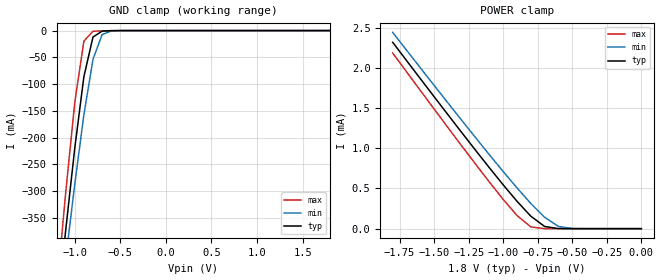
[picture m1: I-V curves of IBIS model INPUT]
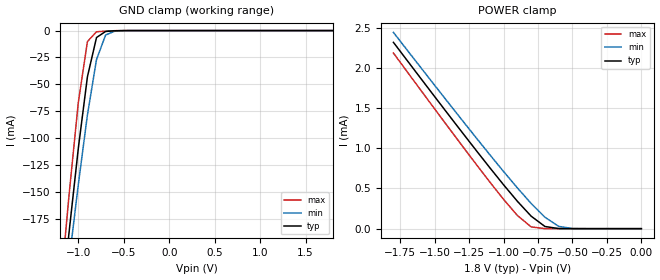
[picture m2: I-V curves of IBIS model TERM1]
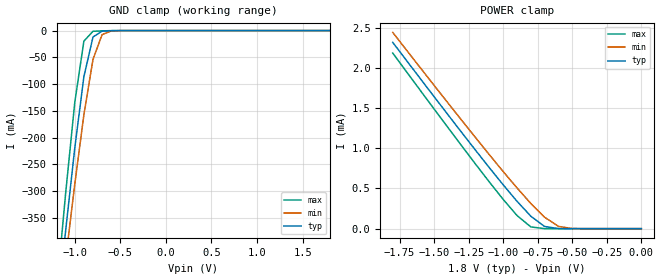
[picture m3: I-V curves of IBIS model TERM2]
|   PERICOM SEMICONDUCTOR CORP
|   IBIS Model of PI4MSD5V9545A
|   Product Family: 4MSD
|   TSSOP-20 (L) Package
[IBIS Ver] 3.2
[Comment char] |_char
[File Name] pi4msd5v9545a_l_18v.ibs
[File Rev] 1.0
[Source] File originated at Pericom Semiconductor Corp.
[Date] 09/07/17
[Disclaimer] (C) Copyright PERICOM Semiconductor Corporation
   All rights reserved
  Pericom Semiconductor Corporation hereby grants the user of
  this IBIS model a non-exclusive, nontransferable license to
  use this IBIS model under the following terms.
  This IBIS model is provided on an "AS IS" basis and Pericom
  makes absolutely no warranty with respect to the information
  contained herein. PERICOM DISCLAIMS AND CUSTOMER WAIVES ALL
  WARRANTIES, EXPRESSED OR IMPLIED, INCLUDING WARRANTIES OF
  MERCHANTABILITY OR FITNESS FOR A PARTICULAR PURPOSE. The
  entire risk as to quality and performance is with the customer.
  Accordingly, in no event shall the company be liable for any
  damages, whether in contract or tort, including any lost
  profits or other incidental, consequential, exemplary, or
  punitive damages arising out of the use or application of the
  IBIS model provided in this package. Further, Pericom reserves
  the right to make changes without notice to any product herein
  to improve reliability, function, or design. Pericom does not
  convey any license under patent rights or any other intellectual
  property rights, including those of third parties.
  The user is granted this license only to use the IBIS model
  and is not granted rights to sell, load, rent, lease or license
  the IBIS model in whole or in part, or in modified form to anyone
  other than user. User may modify the IBIS model to suit its specific
  application but rights to derivative works and such modifications
  shall belong to Pericom.
  Pericom is not obligated to provide maintenance or support
  for the licensed IBIS model.
  Contact Pericom at ATTN: APPLICATION ENGINEERING / IBIS MODELS
  2380 Bering Drive, San Jose, CA 95131
[Component] PI4MSD5V9545A
[Manufacturer] Pericom Semiconductor Corp.
[Package]
| variable   typ   min   max
R_pkg   0.03869ohm   0.03668ohm   0.04069ohm
L_pkg   2.64482nH   2.06962nH   3.22001nH
C_pkg   0.19279pF   0.15543pF   0.23014pF
[Pin] signal_name   model_name   R_pin   L_pin   C_pin
1   A0   INPUT   0.04069   3.22001nH   0.23014pF
2   A1   INPUT   0.03969   2.93241nH   0.21146pF
3   _RESET   INPUT   0.03869   2.64482nH   0.19279pF
4   _INT0   INPUT   0.03768   2.35722nH   0.17411pF
5   SD0   TERM1   0.03668   2.06962nH   0.15543pF
6   SC0   TERM1   0.03668   2.06962nH   0.15543pF
7   _INT1   INPUT   0.03768   2.35722nH   0.17411pF
8   SD1   TERM1   0.03869   2.64482nH   0.19279pF
9   SC1   TERM1   0.03969   2.93241nH   0.21146pF
10   GND   GND   0.04069   3.22001nH   0.23014pF
11   _INT2   INPUT   0.04069   3.22001nH   0.23014pF
12   SD2   TERM1   0.03969   2.93241nH   0.21146pF
13   SC2   TERM1   0.03869   2.64482nH   0.19279pF
14   _INT3   INPUT   0.03768   2.35722nH   0.17411pF
15   SD3   TERM1   0.03668   2.06962nH   0.15543pF
16   SC3   TERM1   0.03668   2.06962nH   0.15543pF
17   _INT   INPUT   0.03768   2.35722nH   0.17411pF
18   SCL   TERM2   0.03869   2.64482nH   0.19279pF
19   SDA   TERM2   0.03969   2.93241nH   0.21146pF
20   VCC   POWER   0.04069   3.22001nH   0.23014pF
[Series Switch Groups]
On 1 /
Off 2 3 4 /
[Series Pin Mapping]   pin_2   model_name  function_table_group
6   18   SWITCH1   1
5   19   SWITCH1   1
9   18   SWITCH1   2
8   19   SWITCH1   2
13   18   SWITCH1   3
12   19   SWITCH1   3
16   18   SWITCH1   4
15   19   SWITCH1   4
|   Model SWITCH1
[Model] SWITCH1
Model_type Series_switch
| variable   typ   min   max
C_comp   7.10pF   7.08pF   7.12pF
[Voltage Range]   1.8000V   1.6200V   1.9800V
[GND Clamp Reference]   0.0000V   0.0000V   0.0000V
[POWER Clamp Reference]   1.8000V   1.6200V   1.9800V
[Temperature Range]   25   85   -40
[On]
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[OFF]
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| Models and submodels in the file (4): INPUT (Input), SWITCH1 (Series_switch), TERM1 (Terminator), TERM2 (Terminator)
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|   Model INPUT
[Model] INPUT
Model_type Input
Vinl = 540mV
Vinh = 1.26V
| variable   typ   min   max
C_comp   4.45pF   4.44pF   4.46pF
[Voltage Range]   1.8000V   1.6200V   1.9800V
[GND Clamp Reference]   0.0000V   0.0000V   0.0000V
[POWER Clamp Reference]   1.8000V   1.6200V   1.9800V
[Temperature Range]   25   85   -40
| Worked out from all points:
|   GND clamp passes 1 mA (typ) near -0.70 V on its own axis
|   POWER clamp passes 1 mA (typ) near -1.21 V on its own axis
[GND Clamp]
| Voltage   I(typ)   I(min)   I(max)
-1.8V     -1.564A    -1.492A    -1.669A
-1.2V     -536.3mA   -573.9mA   -488.8mA
-1.1V     -373.8mA   -427.8mA   -304mA
-1V       -219.8mA   -287.2mA   -134.4mA
-900mV    -86.22mA   -157.4mA   -19.74mA
-800mV    -12.06mA   -53.77mA   -1.311mA
-700mV    -1.032mA   -7.522mA   -526.9uA
-600mV    -210.6uA   -734.5uA   -129.9uA
1.8V      68.64pA    148.9pA    67.17pA
[POWER Clamp]   |Note: Vtable = Vcc - Voutput
| Voltage   I(typ)   I(min)   I(max)
-1.8V     2.317mA    2.441mA    2.184mA
-1.4V     1.417mA    1.564mA    1.257mA
-1.1V     757.6uA    919.3uA    579.7uA
-1V       544.9uA    710.2uA    363.8uA
-900mV    340.5uA    506.6uA    163.7uA
-800mV    155.1uA    313.2uA    21.83uA
-700mV    27.01uA    141.6uA    235.7nA
-600mV    852.4nA    28.01uA    1.729nA
-500mV    17.68nA    1.596uA    108.9pA
0V        68.64pA    88.42pA    75.24pA
|   Model TERM1
[Model] TERM1
Model_type Terminator
| variable   typ   min   max
C_comp   2.65pF   2.64pF   2.66pF
[Voltage Range]   1.8000V   1.6200V   1.9800V
[GND Clamp Reference]   0.0000V   0.0000V   0.0000V
[POWER Clamp Reference]   1.8000V   1.6200V   1.9800V
[Temperature Range]   25   85   -40
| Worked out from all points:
|   GND clamp passes 1 mA (typ) near -0.70 V on its own axis
|   POWER clamp passes 1 mA (typ) near -1.21 V on its own axis
[GND Clamp]
| Voltage   I(typ)   I(min)   I(max)
-1.8V     -779.5mA   -743.6mA   -831.9mA
-1.2V     -267.2mA   -286mA     -243.4mA
-1.1V     -186.2mA   -213.2mA   -151.2mA
-1V       -109.4mA   -143.1mA   -66.79mA
-900mV    -42.98mA   -78.43mA   -10.22mA
-800mV    -6.45mA    -26.94mA   -1.105mA
-700mV    -805uA     -4.15mA    -477.3uA
-600mV    -185.9uA   -544.9uA   -115.7uA
1.8V      37.5pA     93.35pA    36.54pA
[POWER Clamp]   |Note: Vtable = Vcc - Voutput
| Voltage   I(typ)   I(min)   I(max)
-1.8V     2.317mA    2.441mA    2.184mA
-1.4V     1.417mA    1.564mA    1.257mA
-1.1V     757.6uA    919.3uA    579.7uA
-1V       544.9uA    710.2uA    363.8uA
-900mV    340.5uA    506.6uA    163.7uA
-800mV    155.1uA    313.2uA    21.83uA
-700mV    27.01uA    141.6uA    235.6nA
-600mV    852.4nA    28.01uA    1.684nA
-500mV    17.64nA    1.596uA    65.36pA
0V        37.5pA     37.78pA    41.21pA
|   Model TERM2
[Model] TERM2
Model_type Terminator
| variable   typ   min   max
C_comp   4.45pF   4.44pF   4.46pF
[Voltage Range]   1.8000V   1.6200V   1.9800V
[GND Clamp Reference]   0.0000V   0.0000V   0.0000V
[POWER Clamp Reference]   1.8000V   1.6200V   1.9800V
[Temperature Range]   25   85   -40
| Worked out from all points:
|   GND clamp passes 1 mA (typ) near -0.70 V on its own axis
|   POWER clamp passes 1 mA (typ) near -1.21 V on its own axis
[GND Clamp]
| Voltage   I(typ)   I(min)   I(max)
-1.8V     -1.564A    -1.492A    -1.669A
-1.2V     -536.3mA   -573.9mA   -488.8mA
-1.1V     -373.8mA   -427.8mA   -304mA
-1V       -219.8mA   -287.2mA   -134.4mA
-900mV    -86.22mA   -157.4mA   -19.74mA
-800mV    -12.06mA   -53.77mA   -1.311mA
-700mV    -1.032mA   -7.522mA   -526.9uA
-600mV    -210.6uA   -734.5uA   -129.9uA
1.8V      68.64pA    148.9pA    67.17pA
[POWER Clamp]   |Note: Vtable = Vcc - Voutput
| Voltage   I(typ)   I(min)   I(max)
-1.8V     2.317mA    2.441mA    2.184mA
-1.4V     1.417mA    1.564mA    1.257mA
-1.1V     757.6uA    919.3uA    579.7uA
-1V       544.9uA    710.2uA    363.8uA
-900mV    340.5uA    506.6uA    163.7uA
-800mV    155.1uA    313.2uA    21.83uA
-700mV    27.01uA    141.6uA    235.7nA
-600mV    852.4nA    28.01uA    1.729nA
-500mV    17.68nA    1.596uA    108.9pA
0V        68.64pA    88.42pA    75.24pA
